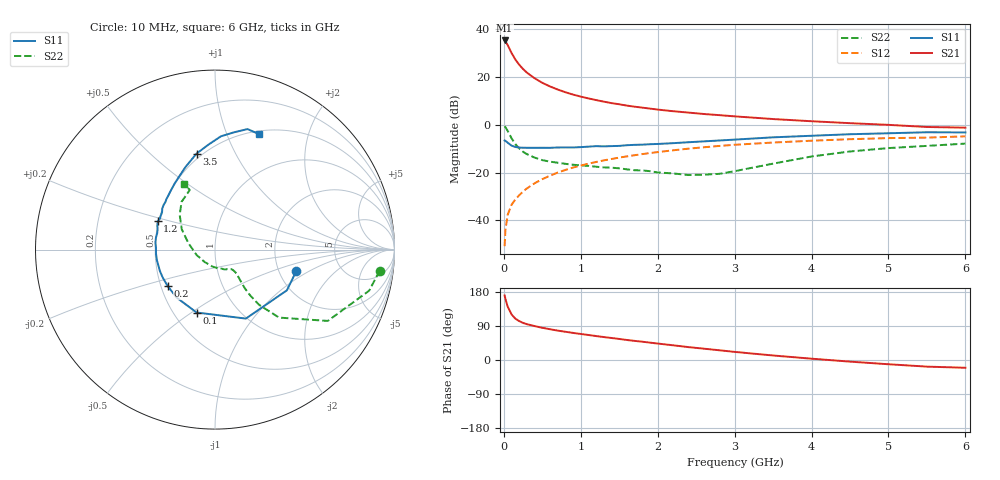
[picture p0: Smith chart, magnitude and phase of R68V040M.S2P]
! SIEMENS Small Signal Semiconductors
! BFR193
! Si NPN RF Bipolar Junction Transistor in SOT23
! VCE = 8 V  IC = 40 mA
! Common Emitter S-Parameters:  May  1996
# GHz  S  MA  R  50
!  f  S11  S21  S12  S22
! GHz  MAG  ANG  MAG  ANG  MAG  ANG  MAG  ANG
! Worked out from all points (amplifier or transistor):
!   36 points, 10 MHz to 6 GHz, reference 50 ohm
!   highest |S21| = 35.2 dB at 10 MHz (marker M1)
!   |S21| within 3 dB of that: start of sweep to 66.35 MHz
!   unconditionally stable (mu >= 1): 473.2 MHz to 2.155 GHz
!   at 250 MHz: K = 0.91, MSG = 25.6 dB, |S12| = -27.9 dB
!   at 1.4 GHz: K = 1.02, MAG = 10.7 dB, |S12| = -14.3 dB
!   at 6 GHz: K = 0.95, MSG = 1.8 dB, |S12| = -4.9 dB
!   S11 on the Smith chart (normalised r, x): 10 MHz: 2.48, -0.77; 100 MHz: 0.65, -0.52; 200 MHz: 0.54, -0.25; 1.2 GHz: 0.49, +0.18; 3.5 GHz: 0.47, +0.71; 6 GHz: 0.53, +1.31
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0.01  0.4682 -14.9  57.51 170.2  0.0029 80.3  0.9247 -7.3
0.02  0.4604 -29.5  55.24 161.7  0.0062 78.4  0.8891 -14.9
0.05  0.4211 -65.9  46.06 140.7  0.0131 69.8  0.7436 -32.3
0.1  0.3652 -106.3  31.58 120.3  0.0212 66.7  0.5206 -46.7
0.15  0.3423 -128.6  22.95 109.1  0.0275 66.5  0.3932 -51.4
0.2  0.333 -142.4  17.9 102.6  0.0336 68.6  0.3199 -52.5
0.25  0.3303 -151.5  14.51 97.9  0.0402 70.0  0.2715 -52.3
0.3  0.3294 -158.7  12.24 94.5  0.0467 71.1  0.2425 -51.5
0.4  0.329 -169.4  9.336 89.5  0.0598 71.8  0.2053 -49.7
0.5  0.3295 -176.0  7.488 85.0  0.0729 72.3  0.1818 -48.3
0.6  0.3288 178.5  6.297 81.2  0.0861 71.7  0.1692 -48.0
0.8  0.3357 168.7  4.765 74.5  0.1134 70.2  0.1523 -48.8
0.9  0.3346 164.6  4.257 71.5  0.1272 69.3  0.1456 -49.3
1.1  0.348 157.5  3.543 66.0  0.1534 67.2  0.1377 -53.5
1.2  0.3564 153.6  3.266 63.2  0.1665 66.0  0.1323 -55.4
1.6  0.3728 142.0  2.505 52.8  0.218 60.4  0.1167 -68.0
2.2  0.4112 126.7  1.912 38.8  0.2918 51.8  0.0959 -98.0
2.8  0.4675 113.3  1.583 25.7  0.3597 42.7  0.094 -149.2
3.5  0.5445 100.9  1.312 11.9  0.424 31.9  0.1537 165.9
4.5  0.6321 87.0  1.076 -4.3  0.4978 18.0  0.2758 135.5
5.5  0.6954 74.9  0.896 -17.5  0.5374 4.3  0.3608 112.9
6  0.6887 69.1  0.867 -20.5  0.5706 0.5  0.4028 115.3
